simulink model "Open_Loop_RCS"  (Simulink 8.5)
settings: Solver=ode4  StartTime=0.0  StopTime=3000  FixedStep=Ts  RelTol=1e-3
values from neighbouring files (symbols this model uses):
  Ave = [    [vehicle_flex34.m]    (also in vehicle_rigid.m)
  Bve = [    [vehicle_flex34.m]    (also in vehicle_rigid.m)
  Cve = [    [vehicle_flex34.m]    (also in vehicle_rigid.m)
  Dve = [    [vehicle_flex34.m]    (also in vehicle_rigid.m)
  Na_max = 0.636/D    (= 72.8802315406)    [Dead_Band_DF.m]    (also in start.m = 0.636/(deadband(1)*d2r); start2.m = 0.636/(deadband(1)*d2r); start3.m = 0.636/(deadband(1)*d2r))
undefined symbols (not defined in the file or in its folder): JSel_ln, Mix, UnitV

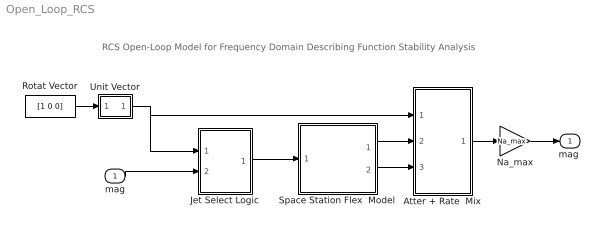
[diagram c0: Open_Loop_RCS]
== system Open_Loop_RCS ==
  note: RCS Open-Loop Model for Frequency Domain Describing Function Stability Analysis
  mag : Inport  PortDimensions=1
  Atter + Rate  Mix : Subsystem
  Jet Select Logic : Subsystem
  Na_max : Gain  Gain=Na_max
  Rotat Vector : Constant  Value=[1 0 0]
  Space Station Flex  Model : Subsystem
  Unit Vector : Subsystem
  "mag " : Outport
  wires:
  Jet Select Logic/1(f(i)) -> Space Station Flex  Model/1(Frcs)
  Space Station Flex  Model/1(att) -> Atter + Rate  Mix/2(atter)
  Space Station Flex  Model/2(wb) -> Atter + Rate  Mix/3(rater)
  mag/1 -> Jet Select Logic/2(mag)
  Unit Vector/1(U) -> Jet Select Logic/1(Udir), Atter + Rate  Mix/1(Udir)
  Rotat Vector/1 -> Unit Vector/1(V)
  Atter + Rate  Mix/1(mag) -> Na_max/1
  Na_max/1 -> "mag "/1

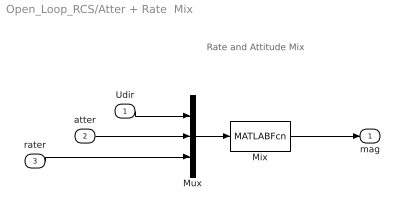
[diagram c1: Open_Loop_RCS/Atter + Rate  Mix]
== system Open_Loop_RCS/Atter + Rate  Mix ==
  note: Rate and Attitude Mix
  Udir : Inport
  atter : Inport  Port=2
  rater : Inport  Port=3
  Mix : MATLABFcn  MATLABFcn=Mix( u(1:3), u(4:6), u(7:9) )  OutputDimensions=1
  Mux : Mux  Inputs="[3  3  3]"
  mag : Outport
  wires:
  rater/1 -> Mux/3
  Mux/1 -> Mix/1
  Udir/1 -> Mux/1
  atter/1 -> Mux/2
  Mix/1 -> mag/1

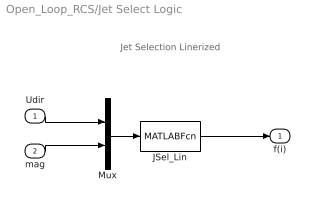
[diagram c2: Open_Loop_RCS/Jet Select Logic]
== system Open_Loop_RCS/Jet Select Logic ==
  note: Jet Selection Linerized
  Udir : Inport
  mag : Inport  Port=2
  JSel_Lin : MATLABFcn  MATLABFcn=JSel_ln( u(1:3), u(4) )  OutputDimensions=nt
  Mux : Mux  Inputs="[3  1]"
  f(i) : Outport
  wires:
  Mux/1 -> JSel_Lin/1
  JSel_Lin/1 -> f(i)/1
  Udir/1 -> Mux/1
  mag/1 -> Mux/2

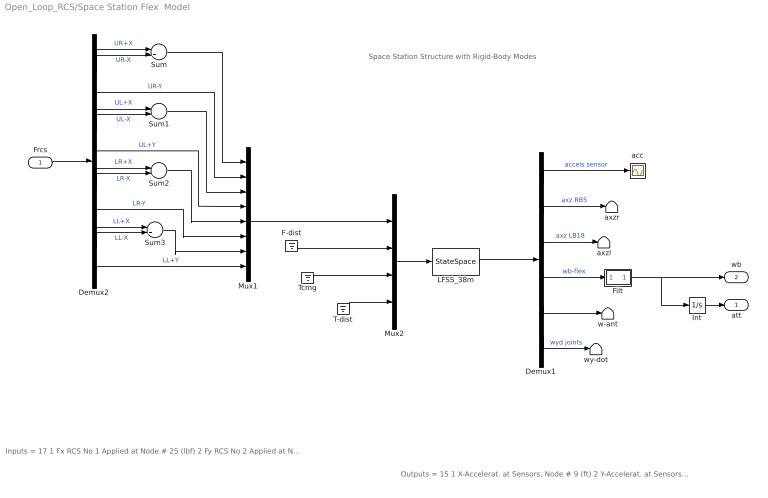
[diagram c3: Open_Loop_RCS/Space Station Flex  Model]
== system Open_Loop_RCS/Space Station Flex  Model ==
  note: Outputs = 15 1 X-Accelerat. at Sensors, Node # 9 (ft) 2 Y-Accelerat. at Sensors, Node # 9 (ft) 3 Z-Accelerat. at Sensors, Node # 9 (ft) 4 X-Accelerat. at Right Boom End, Node # 5 (ft) 5 Z-Accelerat. at Right Boom End, Node # 5 (ft) 6 X-Accelerat. at Left Boom End, Node # 18 (ft) 7 Z-Accelerat. at Left Boom End, Node # 18 (ft) 8 X-Rot. Rate at Sensors, Node # 9 (radian) 9 Y-Rot. Rate at Sensors, Node # 9 (radian) 10 Z-Rot. Rate at Sensors, Node # 9 (radian) 11 X-Rot. Rate at Antena Bot-Left, Node # 24 (radian) 12 Y-Rot. Rate at Antena Bot-Left, Node # 24 (radian) 13 Z-Rot. Rate at Antena Bot-Left, Node # 24 (radian) 14 Y-Rot.Accel. at Right Joint, Node # 7 (radian) 15 Y-Rot.Accel. at Left Joint, Node # 16 (radian)
  note: Inputs = 17 1 Fx RCS No 1 Applied at Node # 25 (lbf) 2 Fy RCS No 2 Applied at Node # 25 (lbf) 3 Fx RCS No 3 Applied at Node # 26 (lbf) 4 Fy RCS No 4 Applied at Node # 26 (lbf) 5 Fx RCS No 5 Applied at Node # 27 (lbf) 6 Fy RCS No 6 Applied at Node # 27 (lbf) 7 Fx RCS No 7 Applied at Node # 28 (lbf) 8 Fy RCS No 8 Applied at Node # 28 (lbf) 9 Fx Disturb. No 9 at Node # 21 (lbf) 10 Fy Disturb. No 10 at Node # 21 (lbf) 11 Fz Disturb. No 11 at Node # 21 (lbf) 12 Torq-x No 1 CMG Applied at Node # 10 (ft-lb) 13 Torq-y No 2 CMG Applied at Node # 10 (ft-lb) 14 Torq-z No 3 CMG Applied at Node # 10 (ft-lb) 15 Torq-x No 4 Gimbal Dist. at Node # 1 (ft-lb) 16 Torq-y No 5 Gimbal Dist. at Node # 1 (ft-lb) 17 Torq-z No 6 Gimbal Dist. at Node # 1 (ft-lb)
  note: Space Station Structure with Rigid-Body Modes
  Frcs : Inport
  Demux1 : Demux  Outputs=[3, 2, 2, 3, 3, 2]
  Demux2 : Demux  Outputs=12
  F-dist : Ground
  Filt : Subsystem
  Int : Integrator
  LFSS_38m : StateSpace  A=Ave  B=Bve  C=Cve  D=Dve  X0=0
  Mux1 : Mux  Inputs=8
  Mux2 : Mux  Inputs=[8, 3, 3, 3]
  Sum{,1..3} (4 alike) : Sum  Inputs=|+-
  T-dist : Ground
  Tcmg : Ground
  acc : Scope
  axzl : Terminator
  axzr : Terminator
  w-ant : Terminator
  wy-dot : Terminator
  att : Outport
  wb : Outport  Port=2
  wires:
  Demux1/6 -> wy-dot/1  "wyd joints"
  Demux1/5 -> w-ant/1
  T-dist/1 -> Mux2/4
  F-dist/1 -> Mux2/2
  Demux1/3 -> axzl/1  "axz LB18"
  Demux1/2 -> axzr/1  "axz RB5"
  Tcmg/1 -> Mux2/3
  Demux1/4 -> Filt/1(I)  "wb-flex"
  Demux1/1 -> acc/1  "accels sensor"
  LFSS_38m/1 -> Demux1/1
  Mux2/1 -> LFSS_38m/1
  Mux1/1 -> Mux2/1
  Frcs/1 -> Demux2/1
  Demux2/6 -> Mux1/4  "UL+Y"
  Demux2/9 -> Mux1/6  "LR-Y"
  Demux2/12 -> Mux1/8  "LL+Y"
  Demux2/3 -> Mux1/2  "UR-Y"
  Demux2/1 -> Sum/1  "UR+X"
  Demux2/2 -> Sum/2  "UR-X"
  Sum/1 -> Mux1/1
  Demux2/4 -> Sum1/1  "UL+X"
  Demux2/5 -> Sum1/2  "UL-X"
  Sum1/1 -> Mux1/3
  Demux2/7 -> Sum2/1  "LR+X"
  Demux2/8 -> Sum2/2  "LR-X"
  Demux2/10 -> Sum3/1  "LL+X"
  Demux2/11 -> Sum3/2  "LL-X"
  Sum3/1 -> Mux1/7
  Sum2/1 -> Mux1/5
  Int/1 -> att/1
  Filt/1(O) -> wb/1, Int/1

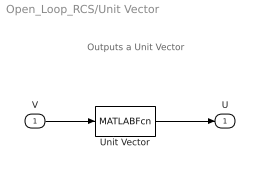
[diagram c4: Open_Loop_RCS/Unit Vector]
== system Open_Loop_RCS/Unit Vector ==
  note: Outputs a Unit Vector
  V : Inport
  Unit Vector : MATLABFcn  MATLABFcn=UnitV( u(1:3) )  OutputDimensions=3
  U : Outport
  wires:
  Unit Vector/1 -> U/1
  V/1 -> Unit Vector/1

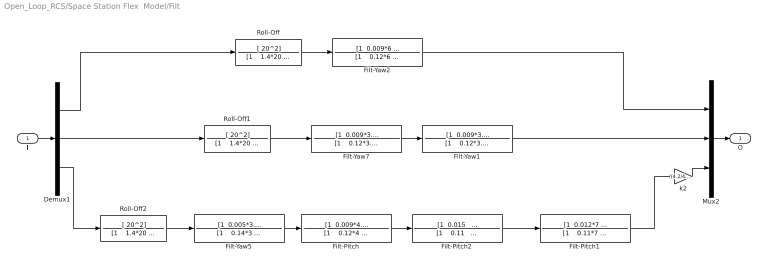
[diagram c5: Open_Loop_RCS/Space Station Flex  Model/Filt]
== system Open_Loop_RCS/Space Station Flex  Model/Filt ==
  I : Inport
  Demux1 : Demux  Outputs=3
  Filt-Pitch : TransferFcn  Numerator="[1  0.009*4.6   4.4^2]"  Denominator="[1    0.12*4    4.2^2]"
  Filt-Pitch1 : TransferFcn  Numerator="[1  0.012*7   6.85^2]"  Denominator="[1    0.11*7    6.85^2]"
  Filt-Pitch2 : TransferFcn  Numerator="[1  0.015   1.14^2]"  Denominator="[1    0.11    1.14^2]"
  Filt-Yaw1 : TransferFcn  Numerator="[1  0.009*3.9   3.93^2]"  Denominator="[1    0.12*3.9    3.93^2]"
  Filt-Yaw2 : TransferFcn  Numerator="[1  0.009*6   5.85^2]"  Denominator="[1    0.12*6    5.85^2]"
  Filt-Yaw5 : TransferFcn  Numerator="[1  0.005*3.1   3.09^2]"  Denominator="[1    0.14*3    3^2]"
  Filt-Yaw7 : TransferFcn  Numerator="[1  0.009*3.5   3.5^2]"  Denominator="[1    0.12*3.5    3.5^2]"
  Mux2 : Mux  Inputs=3
  Roll-Off : TransferFcn  Numerator=[ 20^2]  Denominator="[1    1.4*20    20^2]"
  Roll-Off1 : TransferFcn  Numerator=[ 20^2]  Denominator="[1    1.4*20    20^2]"
  Roll-Off2 : TransferFcn  Numerator=[ 20^2]  Denominator="[1    1.4*20    20^2]"
  k2 : Gain  Gain=(4.2/4.4)*(3/3.09)
  O : Outport
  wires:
  I/1 -> Demux1/1
  Mux2/1 -> O/1
  Demux1/1 -> Roll-Off/1
  Demux1/3 -> Roll-Off2/1
  Demux1/2 -> Roll-Off1/1
  Roll-Off/1 -> Filt-Yaw2/1
  Roll-Off2/1 -> Filt-Yaw5/1
  Roll-Off1/1 -> Filt-Yaw7/1
  Filt-Yaw5/1 -> Filt-Pitch/1
  Filt-Pitch/1 -> Filt-Pitch2/1
  k2/1 -> Mux2/3
  Filt-Yaw7/1 -> Filt-Yaw1/1
  Filt-Yaw1/1 -> Mux2/2
  Filt-Yaw2/1 -> Mux2/1
  Filt-Pitch1/1 -> k2/1
  Filt-Pitch2/1 -> Filt-Pitch1/1
